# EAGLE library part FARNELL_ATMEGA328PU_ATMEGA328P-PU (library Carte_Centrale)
8-bit Microcontroller with In-System Programmable Flash
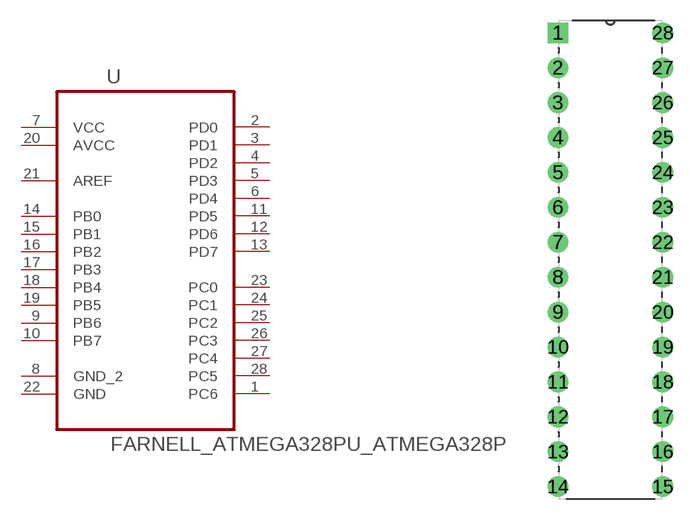
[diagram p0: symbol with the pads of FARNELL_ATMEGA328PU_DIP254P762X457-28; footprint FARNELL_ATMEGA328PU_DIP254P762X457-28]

Designator prefix U

## FARNELL_ATMEGA328PU_ATMEGA328P-PU (MPN: ATMEGA328P-PU; OC_FARNELL: 1715487; OC_NEWARK: 68T2944; PACKAGE: PDIP-28; SUPPLIER: Atmel)  [FARNELL_ATMEGA328PU_DIP254P762X457-28]
1  PC6
2  PD0
3  PD1
4  PD2
5  PD3
6  PD4
7  VCC  pwr
8  GND_2  pas
9  PB6
10  PB7
11  PD5
12  PD6
13  PD7
14  PB0
15  PB1
16  PB2
17  PB3
18  PB4
19  PB5
20  AVCC  pwr
21  AREF  in
22  GND  pas
23  PC0
24  PC1
25  PC2
26  PC3
27  PC4
28  PC5

## Footprint FARNELL_ATMEGA328PU_DIP254P762X457-28 (pad centres in mm)
drill 0.991 square: 1 -7.62,33.02
drill 0.991: 2 -7.62,30.48; 3 -7.62,27.94; 4 -7.62,25.4; 5 -7.62,22.86; 6 -7.62,20.32; 7 -7.62,17.78; 8 -7.62,15.24; 9 -7.62,12.7; 10 -7.62,10.16; 11 -7.62,7.62; 12 -7.62,5.08; 13 -7.62,2.54; 14 -7.62,0; 15 0,0; 16 0,2.54; 17 0,5.08; 18 0,7.62; 19 0,10.16; 20 0,12.7; 21 0,15.24; 22 0,17.78; 23 0,20.32; 24 0,22.86; 25 0,25.4; 26 0,27.94; 27 0,30.48; 28 0,33.02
